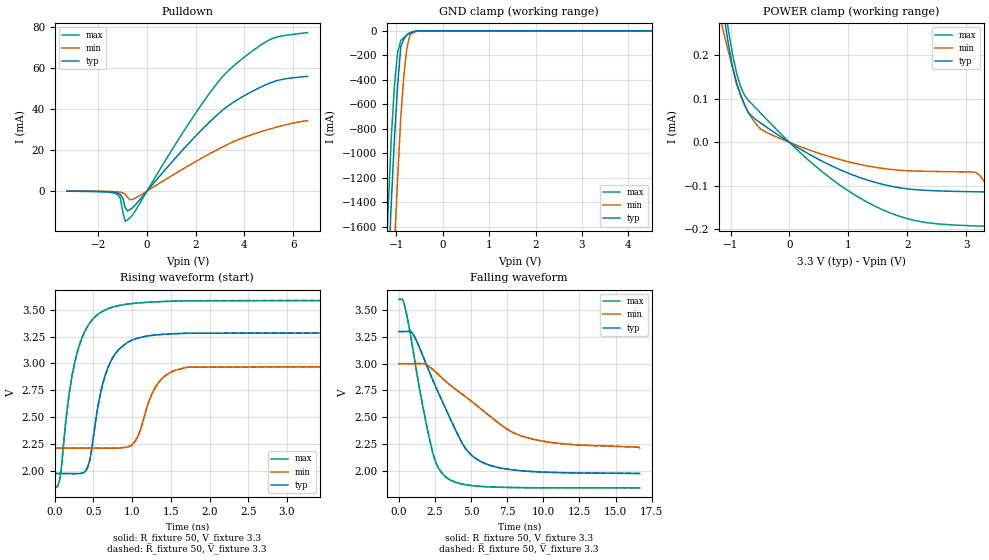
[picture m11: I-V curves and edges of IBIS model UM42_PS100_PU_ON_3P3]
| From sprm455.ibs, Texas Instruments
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|   Model Cell UM42_PS100_PU_ON_3P3
|IDG09_OUM42_PS100_PU_ON_3P3
[Model]   UM42_PS100_PU_ON_3P3
Model_type   I/O_open_drain
Polarity   Non-Inverting
Enable   Active-Low
Vinl =  0.8V
Vinh =  2V
Cref =  15pF
Rref =  100.00M
Vref =  0V
Vmeas =  1.65
C_comp   4.770p   4.586p   5.631p
[Model Spec]
Vinl   0.8V   0.8V   0.8V
Vinh   2V   2V   2V
[Temperature Range]   25   125   -40
[Voltage Range]   3.3   3   3.6
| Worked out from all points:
|   slope of the pulldown table from 0 to 0.495 V, typ, clamps not added: 71.1 ohm
|   GND clamp passes 1 mA (typ) near -0.51 V on its own axis
|   POWER clamp passes 1 mA (typ) near -1.78 V on its own axis
|   rising waveform, R_fixture 50, V_fixture 3.3: 20-80 % time 249ps typ, 264ps min, 250ps max; typ from 1.97 V to 3.3 V
|   rising waveform, R_fixture 50, V_fixture 3.3: 20-80 % time 249ps typ, 264ps min, 250ps max; typ from 1.97 V to 3.3 V
|   falling waveform, R_fixture 50, V_fixture 3.3: 20-80 % time 2.69ns typ, 4.54ns min, 1.47ns max; typ from 3.3 V to 1.97 V
|   falling waveform, R_fixture 50, V_fixture 3.3: 20-80 % time 2.69ns typ, 4.54ns min, 1.47ns max; typ from 3.3 V to 1.97 V
| Nom Voltages:
|   VDD=1.1, VDDS=3.3, VSS=0, VSSS=0
| Min Voltages:
|   VDD=1, VDDS=3, VSS=0, VSSS=0
| Max Voltages:
|   VDD=1.2, VDDS=3.6, VSS=0, VSSS=0
[POWER_clamp]
|   voltage   I(typ)   I(min)   I(max)
-3.3V     2.696mA    1.572mA    4.068mA
-1.167V   346.5uA    280.4uA    410.2uA
-1.1V     280.7uA    242.8uA    316.3uA
-1.033V   222.7uA    206.6uA    254.9uA
-900mV    135.1uA    138.3uA    160uA
-700mV    69.06uA    68.48uA    97.2uA
-500mV    45.48uA    32.08uA    68.8uA
33.33mV   -2.83uA    -1.784uA   -4.359uA
900mV     -65.25uA   -41.06uA   -102.3uA
1.633V    -98.04uA   -60.66uA   -157.8uA
3.1V      -113.4uA   -67.98uA   -191.7uA
3.3V      -113.8uA   -88.42uA   -192.6uA
[Pulldown]
|   voltage   I(typ)   I(min)   I(max)
-3.3V     -125.5uA   -69.78uA   -154uA
-1.3V     -854.4uA   -377.5uA   -1.265mA
-1.1V     -1.818mA   -637.5uA   -3.604mA
-1V       -3.545mA   -939.1uA   -10.26mA
-900mV    -8.267mA   -1.615mA   -14.87mA
-800mV    -9.812mA   -3.181mA   -14.12mA
-700mV    -9.167mA   -4.347mA   -13.12mA
-500mV    -7.047mA   -3.656mA   -10mA
1.7V      23.11mA    12.3mA     32.76mA
3.2V      40.42mA    22.07mA    57.19mA
5V        52.57mA    30.11mA    73.74mA
6.6V      56.07mA    34.37mA    77.47mA
[GND_clamp]
|   voltage   I(typ)   I(min)   I(max)
-3.3V     -22.64A    -23.49A    -22.17A
-1.233V   -2.55A     -3.487A    -2.002A
-1.167V   -1.958A    -2.887A    -1.417A
-1.1V     -1.378A    -2.296A    -853.3mA
-1.033V   -864.3mA   -1.736A    -435.2mA
-966.7mV  -448mA     -1.207A    -177.3mA
-900mV    -129.5mA   -710.5mA   -79.4mA
-833.3mV  -68.49mA   -365.9mA   -55.06mA
-766.7mV  -30.59mA   -139.2mA   -33.98mA
-700mV    -15.85mA   -30.61mA   -16.17mA
-366.7mV  -134.1uA   -202.4uA   -197.3uA
6.6V      0A         0A         0A
[Ramp]
| variable   typ   min   max
dV/dt_f 0.79655743/2.6911613n 0.47376059/4.5465281n  1.0572194/1.4701449n
dV/dt_r  16.69129m/0.12526949n 12.513366m/0.1852733n 19.539301m/0.10354131n
R_load = 50
[Rising Waveform]
R_fixture = 50
V_fixture = 3.3
V_fixture_min = 3
V_fixture_max = 3.6
|   time   V(typ)   V(min)   V(max)
0s        1.974V     2.211V     1.84V
66.54ps   1.974V     2.212V     1.931V
191.4ps   1.974V     2.212V     2.744V
350.1ps   1.977V     2.212V     3.237V
452ps     2.1V       2.211V     3.377V
652.4ps   2.891V     2.211V     3.5V
940.6ps   3.197V     2.221V     3.554V
1.349ns   3.269V     2.83V      3.576V
1.712ns   3.282V     2.965V     3.585V
16.67ns   3.3V       3V         3.6V
[Rising Waveform]
R_fixture = 50
V_fixture = 3.3
V_fixture_min = 3
V_fixture_max = 3.6
|   time   V(typ)   V(min)   V(max)
0s        1.974V     2.211V     1.84V
66.54ps   1.974V     2.212V     1.931V
191.4ps   1.974V     2.212V     2.744V
350.1ps   1.977V     2.212V     3.237V
452ps     2.1V       2.211V     3.377V
652.4ps   2.891V     2.211V     3.5V
940.6ps   3.197V     2.221V     3.554V
1.349ns   3.269V     2.83V      3.576V
1.712ns   3.282V     2.965V     3.585V
16.67ns   3.3V       3V         3.6V
[Falling Waveform]
R_fixture = 50
V_fixture = 3.3
V_fixture_min = 3
V_fixture_max = 3.6
|   time   V(typ)   V(min)   V(max)
0s        3.3V       3V         3.6V
271.5ps   3.3V       3V         3.593V
493.6ps   3.3V       3V         3.489V
1.031ns   3.266V     3V         3.087V
2.334ns   2.853V     2.948V     2.176V
3.271ns   2.57V      2.833V     1.94V
4.743ns   2.186V     2.678V     1.867V
6.407ns   2.046V     2.499V     1.849V
9.283ns   1.992V     2.295V     1.842V
16.67ns   1.974V     2.211V     1.84V
[Falling Waveform]
R_fixture = 50
V_fixture = 3.3
V_fixture_min = 3
V_fixture_max = 3.6
|   time   V(typ)   V(min)   V(max)
0s        3.3V       3V         3.6V
271.5ps   3.3V       3V         3.593V
493.6ps   3.3V       3V         3.489V
1.031ns   3.266V     3V         3.087V
2.334ns   2.853V     2.948V     2.176V
3.271ns   2.57V      2.833V     1.94V
4.743ns   2.186V     2.678V     1.867V
6.407ns   2.046V     2.499V     1.849V
9.283ns   1.992V     2.295V     1.842V
16.67ns   1.974V     2.211V     1.84V
